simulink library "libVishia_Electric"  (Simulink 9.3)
settings: Solver=ode45  StartTime=0.0  StopTime=10.0  RelTol=1e-3  EnableMultiTasking=on
undefined symbols (not defined in the file or in its folder): C, Cp, Cs, ctRange, enable_Diode, fnom, gstart, Inom, Lline, n0, n2, nDamping, nHDamping, nIH, nIq, nLs, nPdamping, nRs, pWCstart, Rline, Rps, Rs, RsC, Tmech, Ts, TstepHw, Unom, xh
libraries: powerlib x111, libVishia_Conv x15, libVishia_Ctrl x6, $bdroot x2, lib_T1Blocks_FB x2, Lib_EnvA x1, lib_AngleBlocks x1
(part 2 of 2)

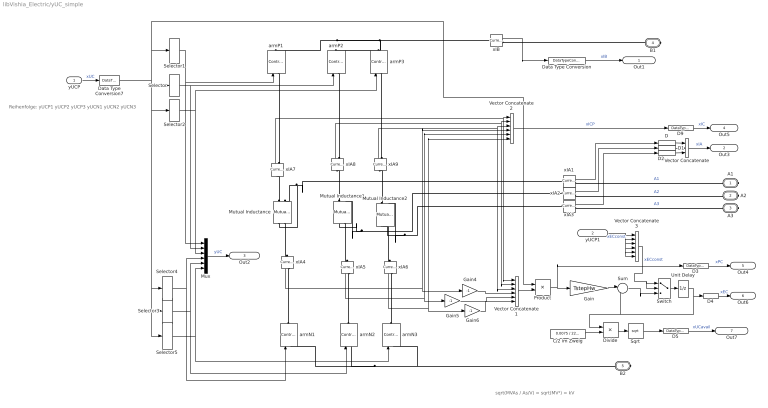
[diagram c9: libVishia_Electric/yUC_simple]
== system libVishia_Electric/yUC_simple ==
  note: sqrt(MVAs / As/V) = sqrt(MV²) = kV
  note: Reihenfolge: yUCP1 yUCP2 yUCP3 yUCN1 yUCN2 yUCN3
  yUCP : Inport  OutDataTypeStr=single  PortDimensions=6  SampleTime=TstepHw
  yUCP1 : Inport  Port=2  OutDataTypeStr=single  PortDimensions=1  SampleTime=TstepHw
  C/2 im Zweig : Constant  Value=0.0075 / 22 / 2
  D{,1..5,9} (7 alike) : DataTypeConversion  OutDataTypeStr=single
  Data Type Conversion : DataTypeConversion  OutDataTypeStr=single
  Data Type Conversion7 : DataTypeConversion  OutDataTypeStr=double
  Divide : Product  Inputs=*/
  Gain : Gain  Gain=TstepHw
  Gain4 : Gain  Gain=-1
  Gain5 : Gain  Gain=-1
  Gain6 : Gain  Gain=-1
  Mutual Inductance : powerlib/Elements/Mutual Inductance  LConnTagsString=a|b  RConnTagsString=A|B  TypeOfMutual=Two or three windings with equal mutual terms  NumberOfWindings=3  SelfImpedance1=[0.01 2.07e-03]  SelfImpedance2=[ 0.01 2.07e-03]  ThreeWindings=off  SelfImpedance3=[ 1.1 1.1e-03]  MutualImpedance=[0.02 0.43e-03]  InductanceMatrix="[1.0 0.9  0.9 ;  0.9 1.0  0.9;  0.9 0.9 1.0 ] * 1e-3"  ResistanceMatrix="[1.0 0.9  0.9 ;  0.9 1.0  0.9;  0.9 0.9 1.0 ]"  Measurements=None
  Mutual Inductance1 : powerlib/Elements/Mutual Inductance  LConnTagsString=a|b  RConnTagsString=A|B  TypeOfMutual=Two or three windings with equal mutual terms  NumberOfWindings=3  SelfImpedance1=[0.01 2.07e-03]  SelfImpedance2=[ 0.01 2.07e-03]  ThreeWindings=off  SelfImpedance3=[ 1.1 1.1e-03]  MutualImpedance=[0.02 0.43e-03]  InductanceMatrix="[1.0 0.9  0.9 ;  0.9 1.0  0.9;  0.9 0.9 1.0 ] * 1e-3"  ResistanceMatrix="[1.0 0.9  0.9 ;  0.9 1.0  0.9;  0.9 0.9 1.0 ]"  Measurements=None
  Mutual Inductance2 : powerlib/Elements/Mutual Inductance  LConnTagsString=a|b  RConnTagsString=A|B  TypeOfMutual=Two or three windings with equal mutual terms  NumberOfWindings=3  SelfImpedance1=[0.01 2.07e-03]  SelfImpedance2=[ 0.01 2.07e-03]  ThreeWindings=off  SelfImpedance3=[ 1.1 1.1e-03]  MutualImpedance=[0.02 0.43e-03]  InductanceMatrix="[1.0 0.9  0.9 ;  0.9 1.0  0.9;  0.9 0.9 1.0 ] * 1e-3"  ResistanceMatrix="[1.0 0.9  0.9 ;  0.9 1.0  0.9;  0.9 0.9 1.0 ]"  Measurements=None
  Mux : Mux  Inputs=6
  Product : Product
  Selector : Selector  InputPortWidth=6  IndexOptions=Index vector (dialog)  Indices=[2]  OutputSizes=1
  Selector1 : Selector  InputPortWidth=6  IndexOptions=Index vector (dialog)  Indices=[1]  OutputSizes=1
  Selector2 : Selector  InputPortWidth=6  IndexOptions=Index vector (dialog)  Indices=[3]  OutputSizes=1
  Selector3 : Selector  InputPortWidth=6  IndexOptions=Index vector (dialog)  Indices=[5]  OutputSizes=1
  Selector4 : Selector  InputPortWidth=6  IndexOptions=Index vector (dialog)  Indices=[4]  OutputSizes=1
  Selector5 : Selector  InputPortWidth=6  IndexOptions=Index vector (dialog)  Indices=[6]  OutputSizes=1
  Sqrt : Sqrt
  Sum : Sum  Inputs=|-+
  Switch : Switch  Criteria=u2 ~= 0
  Unit Delay : UnitDelay  InitialCondition=pWCstart  SampleTime=TstepHw  HasFrameUpgradeWarning=on
  Vector Concatenate : Concatenate  NumInputs=3
  Vector Concatenate1 : Concatenate  NumInputs=6
  Vector Concatenate2 : Concatenate  NumInputs=6
  Vector Concatenate3 : Concatenate  NumInputs=6
  armN1 : powerlib/Electrical Sources/Controlled Voltage Source  Initialize=on  Source_Type=DC  Amplitude=0  Phase=0  Frequency=0  Measurements=None
  armN2 : powerlib/Electrical Sources/Controlled Voltage Source  Initialize=on  Source_Type=DC  Amplitude=0  Phase=0  Frequency=0  Measurements=None
  armN3 : powerlib/Electrical Sources/Controlled Voltage Source  Initialize=on  Source_Type=DC  Amplitude=0  Phase=0  Frequency=0  Measurements=None
  armP1 : powerlib/Electrical Sources/Controlled Voltage Source  Initialize=on  Source_Type=DC  Amplitude=0  Phase=0  Frequency=0  Measurements=None
  armP2 : powerlib/Electrical Sources/Controlled Voltage Source  Initialize=on  Source_Type=DC  Amplitude=0  Phase=0  Frequency=0  Measurements=None
  armP3 : powerlib/Electrical Sources/Controlled Voltage Source  Initialize=on  Source_Type=DC  Amplitude=0  Phase=0  Frequency=0  Measurements=None
  xIA{1..9} (9 alike) : powerlib/Measurements/Current Measurement  PhasorSimulation=off  OutputType=Complex  PSBequivalent=0
  xIB : powerlib/Measurements/Current Measurement  PhasorSimulation=off  OutputType=Complex  PSBequivalent=0
  A1 : PMIOPort  Tag=PMCPort  Side=Right
  A2 : PMIOPort  Tag=PMCPort  Port=2  Side=Right
  A3 : PMIOPort  Tag=PMCPort  Port=3  Side=Right
  B1 : PMIOPort  Tag=PMCPort  Port=4  Side=Right
  B2 : PMIOPort  Tag=PMCPort  Port=5  Side=Right
  Out1 : Outport  OutDataTypeStr=single  PortDimensions=1  SampleTime=TstepHw
  Out3 : Outport  Port=2  OutDataTypeStr=single  PortDimensions=3  SampleTime=TstepHw
  Out2 : Outport  Port=3  SampleTime=TstepHw
  Out5 : Outport  Port=4  OutDataTypeStr=single  PortDimensions=6  SampleTime=TstepHw
  Out4 : Outport  Port=5  OutDataTypeStr=single  PortDimensions=6  SampleTime=TstepHw
  Out6 : Outport  Port=6  OutDataTypeStr=single  PortDimensions=6  SampleTime=TstepHw
  Out7 : Outport  Port=7  OutDataTypeStr=single  PortDimensions=6
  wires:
  yUCP/1 -> Data Type Conversion7/1  "xUC"
  xIB/1 -> Data Type Conversion/1
  Data Type Conversion/1 -> Out1/1  "xIB"
  Selector1/1 -> Mux/1, armP1/1
  Selector/1 -> armP2/1, Mux/2
  Selector2/1 -> Mux/3, armP3/1
  Selector4/1 -> armN1/1, Mux/4
  Selector3/1 -> armN2/1, Mux/5
  Selector5/1 -> Mux/6, armN3/1
  Mux/1 -> Out2/1  "yUC"
  xIA1/1 -> D/1
  xIA2/1 -> D1/1
  xIA3/1 -> D2/1
  Vector Concatenate/1 -> Out3/1  "xIA"
  D/1 -> Vector Concatenate/1
  D1/1 -> Vector Concatenate/2
  D2/1 -> Vector Concatenate/3
  xIA4/1 -> Gain4/1, Vector Concatenate2/4
  xIA5/1 -> Gain5/1, Vector Concatenate2/5
  D9/1 -> Out5/1  "xIC"
  Product/1 -> Gain/1, D3/1
  D3/1 -> Out4/1  "xPC"
  Data Type Conversion7/1 -> Product/1, Selector1/1, Selector5/1, Selector3/1, Selector4/1, Selector2/1, Selector/1
  D4/1 -> Out6/1  "xEC"
  Divide/1 -> Sqrt/1
  C/2 im Zweig/1 -> Divide/2
  D5/1 -> Out7/1  "xUCavail"
  Sqrt/1 -> D5/1
  Unit Delay/1 -> Divide/1, Sum/2, D4/1
  Gain/1 -> Sum/1
  Sum/1 -> Switch/3
  Vector Concatenate2/1 -> D9/1  "xICP"
  Vector Concatenate1/1 -> Product/2
  xIA7/1 -> Vector Concatenate2/1, Vector Concatenate1/1
  xIA8/1 -> Vector Concatenate2/2, Vector Concatenate1/2
  xIA9/1 -> Vector Concatenate2/3, Vector Concatenate1/3
  Gain6/1 -> Vector Concatenate1/6
  xIA6/1 -> Gain6/1, Vector Concatenate2/6
  Gain5/1 -> Vector Concatenate1/5
  Gain4/1 -> Vector Concatenate1/4
  Switch/1 -> Unit Delay/1
  Vector Concatenate3/1 -> Switch/2, Switch/1  "xECconst"
  yUCP1/1 -> Vector Concatenate3/6, Vector Concatenate3/5, Vector Concatenate3/4, Vector Concatenate3/3, Vector Concatenate3/2, Vector Concatenate3/1  "xECconst"
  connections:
  B2/RConn1 -- armN1/LConn1 -- armN2/LConn1 -- armN3/LConn1
  armP1/RConn1 -- armP2/RConn1 -- xIB/LConn1 -- armP3/RConn1
  B1/RConn1 -- xIB/RConn1
  A1/RConn1 -- xIA1/RConn1  "A1"
  xIA2/RConn1 -- A2/RConn1  "A2"
  A3/RConn1 -- xIA3/RConn1  "A3"
  armP1/LConn1 -- xIA7/RConn1
  armP2/LConn1 -- xIA8/RConn1
  armP3/LConn1 -- xIA9/RConn1
  Mutual Inductance/RConn2 -- xIA4/LConn1
  Mutual Inductance1/RConn2 -- xIA5/LConn1
  Mutual Inductance2/RConn2 -- xIA6/LConn1
  Mutual Inductance/LConn1 -- xIA7/LConn1
  Mutual Inductance1/LConn1 -- xIA8/LConn1
  Mutual Inductance2/LConn1 -- xIA9/LConn1
  Mutual Inductance/RConn1 -- xIA1/LConn1 -- Mutual Inductance/LConn2
  xIA2/LConn1 -- Mutual Inductance1/RConn1 -- Mutual Inductance1/LConn2
  xIA3/LConn1 -- Mutual Inductance2/RConn1 -- Mutual Inductance2/LConn2
  armN1/RConn1 -- xIA4/RConn1
  armN2/RConn1 -- xIA5/RConn1
  armN3/RConn1 -- xIA6/RConn1

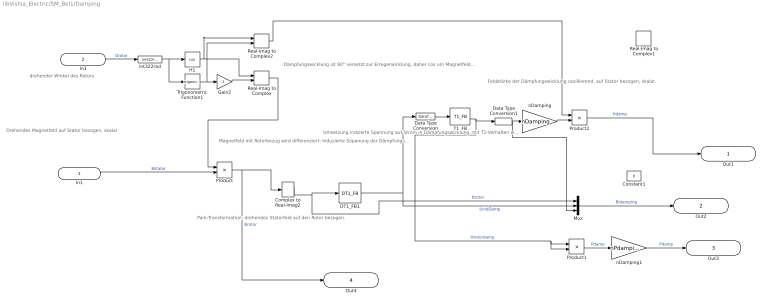
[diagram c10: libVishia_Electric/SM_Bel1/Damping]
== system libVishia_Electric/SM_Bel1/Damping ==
  note: Drehendes Magnetfeld auf Stator bezogen, skalar
  note: drehender Winkel des Rotors
  note: Park-Transformation: drehendes Statorfeld auf den Rotor bezogen.
  note: Magnetfeld mit Rotorbezug wird differenziert: Induzierte Sopanung der Dämpfungswicklung
  note: Umsetzung indzierte Spannung auf Strom in Dämpfungswicklung, mit T1-Verhalten wegen L/R
  note: Dämpfungswicklung ist 90° versetzt zur Erregerwicklung, daher cos um Magnetfeld mit Rotorbezug auf den Stator umzurechnen
  note: Feldstärke der Dämpfungswicklung oszillierend, auf Stator bezogen, skalar.
  In1 : Inport  OutDataTypeStr=single  PortDimensions=1
  In3 : Inport  Port=2  OutDataTypeStr=int32  PortDimensions=1
  Complex to Real-Imag2 : ComplexToRealImag
  Constant1 : Constant  Value=0  OutDataTypeStr=single
  DT1_FB1 : lib_T1Blocks_FB/DT1_FB  T1=0.001  Td=0.01  Tstep=TstepHw
  Data Type Conversion : DataTypeConversion  OutDataTypeStr=double
  Data Type Conversion1 : DataTypeConversion  OutDataTypeStr=single
  Gain2 : Gain  Gain=-1
  H1 : Trigonometry  Operator=cos
  Mux : Mux  Inputs=3
  Product : Product
  Product1 : Product
  Product2 : Product
  Real-Imag to Complex : RealImagToComplex
  Real-Imag to Complex1 : RealImagToComplex
  Real-Imag to Complex2 : RealImagToComplex
  T1_FB : lib_T1Blocks_FB/T1_FB  T1=TsDamping  y0=0  Tstep=TstepHw
  Trigonometric Function1 : Trigonometry
  int322rad : lib_AngleBlocks/int322rad
  nDamping : Gain  Gain=nDamping
  nDamping1 : Gain  Gain=nPdamping
  Out1 : Outport  OutDataTypeStr=single  PortDimensions=1
  Out2 : Outport  Port=2  OutDataTypeStr=single  PortDimensions=3
  Out3 : Outport  Port=3  OutDataTypeStr=double  PortDimensions=1
  Out4 : Outport  Port=4  OutDataTypeStr=single  PortDimensions=1
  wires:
  T1_FB/2 -> Product1/2, Product1/1, Data Type Conversion1/1  "Hrotordamp"
  Gain2/1 -> Real-Imag to Complex/2
  Trigonometric Function1/1 -> Real-Imag to Complex2/2, Gain2/1
  int322rad/1 -> H1/1, Trigonometric Function1/1
  In3/1 -> int322rad/1  "Grotor"
  Product/1 -> Out4/1, Complex to Real-Imag2/1  "Brotor"
  Complex to Real-Imag2/1 -> Mux/1, DT1_FB1/1  "Brotor"
  DT1_FB1/2 -> Data Type Conversion/1, Mux/2  "UindDamp"
  Product2/1 -> Out1/1  "Hdamp"
  H1/1 -> Real-Imag to Complex2/1, Real-Imag to Complex/1
  In1/1 -> Product/2  "Bstator"
  Constant1/1 -> ?
  Mux/1 -> Out2/1  "BIdamping"
  Real-Imag to Complex2/1 -> Product2/1
  Data Type Conversion/1 -> T1_FB/1
  nDamping/1 -> Product2/2
  nDamping1/1 -> Out3/1  "Pdamp"
  Real-Imag to Complex/1 -> Product/1
  Data Type Conversion1/1 -> Mux/3, nDamping/1
  Product1/1 -> nDamping1/1  "Pdamp"

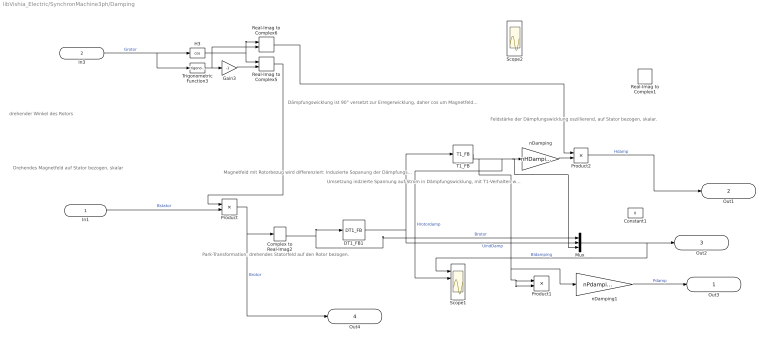
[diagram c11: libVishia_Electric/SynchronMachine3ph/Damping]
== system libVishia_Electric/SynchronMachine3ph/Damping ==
  note: Feldstärke der Dämpfungswicklung oszillierend, auf Stator bezogen, skalar.
  note: Dämpfungswicklung ist 90° versetzt zur Erregerwicklung, daher cos um Magnetfeld mit Rotorbezug auf den Stator umzurechnen
  note: Umsetzung indzierte Spannung auf Strom in Dämpfungswicklung, mit T1-Verhalten wegen L/R
  note: Magnetfeld mit Rotorbezug wird differenziert: Induzierte Sopanung der Dämpfungswicklung
  note: Park-Transformation: drehendes Statorfeld auf den Rotor bezogen.
  note: drehender Winkel des Rotors
  note: Drehendes Magnetfeld auf Stator bezogen, skalar
  In1 : Inport  OutDataTypeStr=double  PortDimensions=1
  In3 : Inport  Port=2  OutDataTypeStr=double  PortDimensions=1
  Complex to Real-Imag2 : ComplexToRealImag
  Constant1 : Constant  Value=0  OutDataTypeStr=single
  DT1_FB1 : libVishia_Ctrl/DT1_FB  T1=0.1  Td=1  Tstep=TstepHw
  Gain3 : Gain  Gain=-1
  H3 : Trigonometry  Operator=cos
  Mux : Mux  Inputs=3
  Product : Product
  Product1 : Product
  Product2 : Product
  Real-Imag to Complex1 : RealImagToComplex
  Real-Imag to Complex5 : RealImagToComplex
  Real-Imag to Complex6 : RealImagToComplex
  Scope1 : Scope  NumInputPorts=4
  Scope2 : Scope  NumInputPorts=4
  T1_FB : libVishia_Ctrl/T1_FB  T1=TsDamping  y0=0  Tstep=TstepHw
  Trigonometric Function3 : Trigonometry
  nDamping : Gain  Gain=nHDamping
  nDamping1 : Gain  Gain=nPdamping
  Out3 : Outport  OutDataTypeStr=double  PortDimensions=1
  Out1 : Outport  Port=2  OutDataTypeStr=double  PortDimensions=1
  Out2 : Outport  Port=3  OutDataTypeStr=double
  Out4 : Outport  Port=4  OutDataTypeStr=double  PortDimensions=1
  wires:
  Real-Imag to Complex5/1 -> Product/1
  nDamping/1 -> Product2/2
  Mux/1 -> Out2/1, Scope1/1  "BIdamping"
  Constant1/1 -> ?
  In1/1 -> Product/2  "Bstator"
  Product2/1 -> Out1/1  "Hdamp"
  DT1_FB1/2 -> Mux/2, T1_FB/1  "UindDamp"
  Complex to Real-Imag2/2 -> Mux/1, DT1_FB1/1  "Brotor"
  Product/1 -> Out4/1, Complex to Real-Imag2/1  "Brotor"
  In3/1 -> H3/1, Trigonometric Function3/1  "Grotor"
  T1_FB/2 -> nDamping/1, Mux/3, Scope1/2, Product1/2, Product1/1, nDamping1/1  "Hrotordamp"
  Trigonometric Function3/1 -> Real-Imag to Complex6/2, Gain3/1
  H3/1 -> Real-Imag to Complex5/1, Real-Imag to Complex6/1
  Gain3/1 -> Real-Imag to Complex5/2
  Real-Imag to Complex6/1 -> Product2/1
  nDamping1/1 -> Out3/1  "Pdamp"
